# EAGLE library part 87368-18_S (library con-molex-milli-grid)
RECEPTACAL
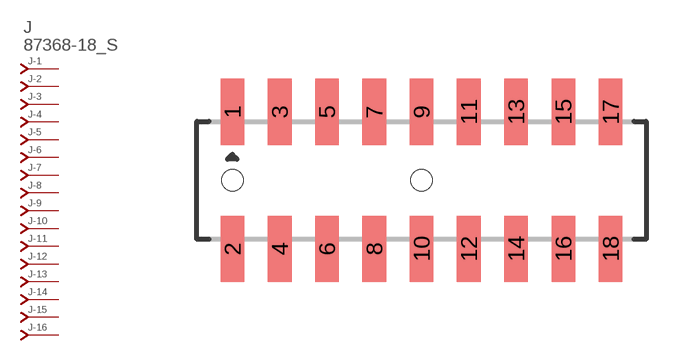
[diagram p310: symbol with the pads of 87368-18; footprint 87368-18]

Designator prefix J; gates -1=J-NV -2=J-N -3=J-N -4=J-N -5=J-N -6=J-N -7=J-N -8=J-N -9=J-N -10=J-N -11=J-N -12=J-N -13=J-N -14=J-N -15=J-N -16=J-N -17=J-N -18=J-N

## 87368-18_S  [87368-18]
1  -1:J  pas
2  -2:J  pas
3  -3:J  pas
4  -4:J  pas
5  -5:J  pas
6  -6:J  pas
7  -7:J  pas
8  -8:J  pas
9  -9:J  pas
10  -10:J  pas
11  -11:J  pas
12  -12:J  pas
13  -13:J  pas
14  -14:J  pas
15  -15:J  pas
16  -16:J  pas
17  -17:J  pas
18  -18:J  pas

## Footprint 87368-18 (pad centres in mm)
RECEPTACAL SMD Dual Row, Side Entry
smd 1 x 2.8: 1 -8,2.9; 2 -8,-2.9; 3 -6,2.9; 4 -6,-2.9; 5 -4,2.9; 6 -4,-2.9; 7 -2,2.9; 8 -2,-2.9; 9 0,2.9; 10 0,-2.9; 11 2,2.9; 12 2,-2.9; 13 4,2.9; 14 4,-2.9; 15 6,2.9; 16 6,-2.9; 17 8,2.9; 18 8,-2.9
hole 0.914 at -8,0
hole 0.914 at 0,0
